ORGANIZATION_BLOCK OB 1
TITLE = "Main Program Sweep (Cycle)"
VERSION : 0.1


VAR_TEMP
  OB1_EV_CLASS : BYTE ;	//Bits 0-3 = 1 (Coming event), Bits 4-7 = 1 (Event class 1)
  OB1_SCAN_1 : BYTE ;	//1 (Cold restart scan 1 of OB 1), 3 (Scan 2-n of OB 1)
  OB1_PRIORITY : BYTE ;	//1 (Priority of 1 is lowest)
  OB1_OB_NUMBR : BYTE ;	//1 (Organization block 1, OB1)
  OB1_RESERVED_1 : BYTE ;	//Reserved for system
  OB1_RESERVED_2 : BYTE ;	//Reserved for system
  OB1_PREV_CYCLE : INT ;	//Cycle time of previous OB1 scan (milliseconds)
  OB1_MIN_CYCLE : INT ;	//Minimum cycle time of OB1 (milliseconds)
  OB1_MAX_CYCLE : INT ;	//Maximum cycle time of OB1 (milliseconds)
  OB1_DATE_TIME : DATE_AND_TIME ;	//Date and time OB1 started
END_VAR
BEGIN
NETWORK
TITLE =

      CALL "GESTIONE CONTATORE" ;
      CALL "MODI MACCHINA" ;
      CALL "FRONTI POS. E NEG." ;
      CALL "COMUNICAZIONE OP" ;
      CALL "COMUNICAZIONE LINEA" ;
      CALL "MANUALI" ;
      CALL "AUTOMATICO" ;
      CALL "CICLO GIOSTRA + DX" ;
      CALL "CICLO GIOSTRA + SX" ;
      CALL "CICLO GIOSTRA - DX" ;
      CALL "CICLO GIOSTRA - SX" ;
      CALL "CICLO MANIP. POSITIVE" ;
      CALL "CICLO MANIP. NEGATIVE" ;
      CALL "CICLO FORMAZIONE PACCHI" ;
      CALL "CICLO CATENE USCITA" ;
      CALL "CICLO CATENE POSITIVE" ;
      CALL "CICLO CATENE NEGATIVE" ;
      CALL "CICLO SVOLGITORE" ;
      CALL "VELOCITA' INVERTER" ;
      CALL "CICLO ROBOT" ;
      CALL "SINCRONIZZAZIONE ASSI" ;
      CALL "ASSE X" ;
      CALL "ASSE Y" ;
      CALL "ASSE Z" ;
      CALL "DIAGNOSTICA" ;
      CALL "COMANDO USCITE" ;
      CALL "Conteggi" ;


NETWORK
TITLE =COMUNICAZIONE CON GLI AZIONAMENTI

//°°°°°°°°°°°°°°°°°°°°°°°°°°°°°°°°°°°°°°°°
//            ASSE X
//________________________________________
      CALL "DPWR_DAT" (
           LADDR                    := W#16#104,
           RECORD                   := P#DB121.DBX0.0 BYTE 8,
           RET_VAL                  := MW   200);
      L     DB121.DBW    8;
      T     PAW  268;
      L     DB121.DBW   10;
      T     PAW  270;
      L     DB121.DBW   12;
      T     PAW  272;
      L     DB121.DBW   14;
      T     PAW  274;
      L     "DB ASSE X".OVERRIDE;
      T     PAW  276;
      L     "DB ASSE X".DAC1;
      T     PAW  278;
      L     "DB ASSE X".DAC2;
      T     PAW  280;
      L     DB121.DBW   22;
      T     PAW  282;
      L     "DB ASSE X".MOMRID;
      T     PAW  284;
      L     "DB ASSE X".PZD10;
      T     PAW  286;
//-------------------------------------
      CALL "DPRD_DAT" (
           LADDR                    := W#16#100,
           RET_VAL                  := MW   202,
           RECORD                   := P#DB121.DBX28.0 BYTE 8);
      L     PEW  264;
      T     DB121.DBW   36;
      L     PEW  266;
      T     DB121.DBW   38;
      L     PEW  268;
      T     DB121.DBW   40;
      L     PEW  270;
      T     DB121.DBW   42;
      L     PEW  272;
      T     DB121.DBW   44;
      L     PEW  274;
      T     "DB ASSE X".ADC1;
      L     PEW  276;
      T     "DB ASSE X".ADC2;
      L     PEW  278;
      T     "DB ASSE X".MRIF1;
      L     PEW  280;
      T     DB121.DBW   52;
      L     PEW  282;
      T     DB121.DBW   54;
//°°°°°°°°°°°°°°°°°°°°°°°°°°°°°°°°°°°°°°°°
//            ASSE Y
//________________________________________
      CALL "DPWR_DAT" (
           LADDR                    := W#16#120,
           RECORD                   := P#DB122.DBX0.0 BYTE 8,
           RET_VAL                  := MW   200);
      L     DB122.DBW    8;
      T     PAW  296;
      L     DB122.DBW   10;
      T     PAW  298;
      L     DB122.DBW   12;
      T     PAW  300;
      L     DB122.DBW   14;
      T     PAW  302;
      L     "DB ASSE Y".OVERRIDE;
      T     PAW  304;
      L     "DB ASSE Y".DAC1;
      T     PAW  306;
      L     "DB ASSE Y".DAC2;
      T     PAW  308;
      L     DB122.DBW   22;
      T     PAW  310;
      L     "DB ASSE Y".MOMRID;
      T     PAW  312;
      L     "DB ASSE Y".PZD10;
      T     PAW  314;
//-------------------------------------
      CALL "DPRD_DAT" (
           LADDR                    := W#16#11C,
           RET_VAL                  := MW   202,
           RECORD                   := P#DB122.DBX28.0 BYTE 8);
      L     PEW  292;
      T     DB122.DBW   36;
      L     PEW  294;
      T     DB122.DBW   38;
      L     PEW  296;
      T     DB122.DBW   40;
      L     PEW  298;
      T     DB122.DBW   42;
      L     PEW  300;
      T     DB122.DBW   44;
      L     PEW  302;
      T     "DB ASSE Y".ADC1;
      L     PEW  304;
      T     "DB ASSE Y".ADC2;
      L     PEW  306;
      T     "DB ASSE Y".MRIF1;
      L     PEW  308;
      T     DB122.DBW   52;
      L     PEW  310;
      T     DB122.DBW   54;
//°°°°°°°°°°°°°°°°°°°°°°°°°°°°°°°°°°°°°°°°
//            ASSE Z
//________________________________________
      CALL "DPWR_DAT" (
           LADDR                    := W#16#13C,
           RECORD                   := P#DB123.DBX0.0 BYTE 8,
           RET_VAL                  := MW   200);
      L     DB123.DBW    8;
      T     PAW  356;
      L     DB123.DBW   10;
      T     PAW  358;
      L     DB123.DBW   12;
      T     PAW  360;
      L     DB123.DBW   14;
      T     PAW  362;
      L     "DB ASSE Z".OVERRIDE;
      T     PAW  364;
      L     "DB ASSE Z".DAC1;
      T     PAW  366;
      L     "DB ASSE Z".DAC2;
      T     PAW  368;
      L     DB123.DBW   22;
      T     PAW  370;
      L     "DB ASSE Z".MOMRID;
      T     PAW  372;
      L     "DB ASSE Z".PZD10;
      T     PAW  374;
//-------------------------------------
      CALL "DPRD_DAT" (
           LADDR                    := W#16#138,
           RET_VAL                  := MW   202,
           RECORD                   := P#DB123.DBX28.0 BYTE 8);
      L     PEW  320;
      T     DB123.DBW   36;
      L     PEW  322;
      T     DB123.DBW   38;
      L     PEW  324;
      T     DB123.DBW   40;
      L     PEW  326;
      T     DB123.DBW   42;
      L     PEW  328;
      T     DB123.DBW   44;
      L     PEW  330;
      T     "DB ASSE Z".ADC1;
      L     PEW  332;
      T     "DB ASSE Z".ADC2;
      L     PEW  334;
      T     "DB ASSE Z".MRIF1;
      L     PEW  336;
      T     DB123.DBW   52;
      L     PEW  338;
      T     DB123.DBW   54;

NETWORK
TITLE =COMUNICAZIONE CON QUADRO LINEA DI TRASPORTO

      CALL "AG_SEND" (
           ACT                      := TRUE,
           ID                       := 1,
           LADDR                    := W#16#154,
           SEND                     := P#DB112.DBX10.0 BYTE 10,
           LEN                      := 10,
           DONE                     := "DB COMUNICAZIONE LINEA".Done,
           ERROR                    := "DB COMUNICAZIONE LINEA".ErrorTrasm,
           STATUS                   := "DB COMUNICAZIONE LINEA".StatusTrasm);
//---------------------------------------
      CALL "AG_RECV" (
           ID                       := 1,
           LADDR                    := W#16#154,
           RECV                     := P#DB112.DBX0.0 BYTE 10,
           NDR                      := "DB COMUNICAZIONE LINEA".NDR,
           ERROR                    := "DB COMUNICAZIONE LINEA".ErrorRic,
           STATUS                   := "DB COMUNICAZIONE LINEA".StatusRic,
           LEN                      := "DB COMUNICAZIONE LINEA".LEN);

NETWORK
TITLE =prove

      SPA   M002;
//°°°°°°°°°°°°°°°°°°°°°°°°°°°°°°°°°°°°°°°°°°//
//    CONTROLLO RICHIESTA ROTAZIONE PINZA   //
//__________________________________________//
      AUF   "DB DATI";
      L     P#26.0;
      LAR1  ;
      L     "DB DATI".PACCHI_DEPOSITATI;
      L     16;
      *I    ;
      +AR1  ;
      L     DBW [AR1,P#0.0];
      L     1;
      ==I   ;
      =     "CR.BR180°";
//===================================
      U     "P.R.PR";
      FP    "CR.RRPP";
      SPBN  M001;
      L     "DB DATI".PACCHI_DEPOSITATI;
      L     1;
      +I    ;
      T     "DB DATI".PACCHI_DEPOSITATI;
M001: NOP   0;
      U     "TRT";
      SPBN  M002;
      L     0;
      T     "DB DATI".PACCHI_DEPOSITATI;
M002: NOP   0;

NETWORK
TITLE =
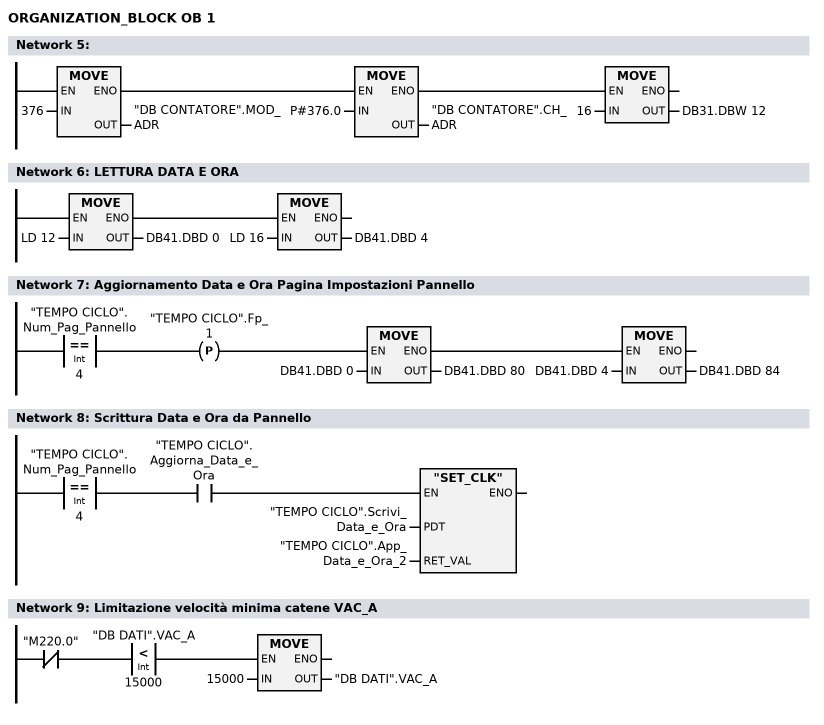
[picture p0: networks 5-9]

      L     376;
      T     "DB CONTATORE".MOD_ADR;
      L     P#376.0;
      T     "DB CONTATORE".CH_ADR;
      L     16;
      T     DB31.DBW   12;
NETWORK
TITLE =LETTURA DATA E ORA

      L     LD    12;
      T     DB41.DBD    0;

      L     LD    16;
      T     DB41.DBD    4;


NETWORK
TITLE =Aggiornamento Data e Ora Pagina Impostazioni Pannello

      L     "TEMPO CICLO".Num_Pag_Pannello;
      L     4;
      ==I   ;
      FP    "TEMPO CICLO".Fp_1;
      SPBN  s07;
      L     DB41.DBD    0;
      T     DB41.DBD   80;
      L     DB41.DBD    4;
      T     DB41.DBD   84;
s07:  NOP   0;

NETWORK
TITLE =Scrittura Data e Ora da Pannello

      L     "TEMPO CICLO".Num_Pag_Pannello;
      L     4;
      ==I   ;
      U     "TEMPO CICLO".Aggiorna_Data_e_Ora;
      SPBN  s08;
      CALL "SET_CLK" (
           PDT                      := "TEMPO CICLO".Scrivi_Data_e_Ora,
           RET_VAL                  := "TEMPO CICLO".App_Data_e_Ora_2);
      NOP   0;
s08:  NOP   0;
NETWORK
TITLE =Limitazione velocità minima catene VAC_A



      UN    "M220.0";
      U(    ;
      L     "DB DATI".VAC_A;
      L     15000;
      <I    ;
      )     ;
      SPBNB _001;
      L     15000;
      T     "DB DATI".VAC_A;
_001: NOP   0;
END_ORGANIZATION_BLOCK

